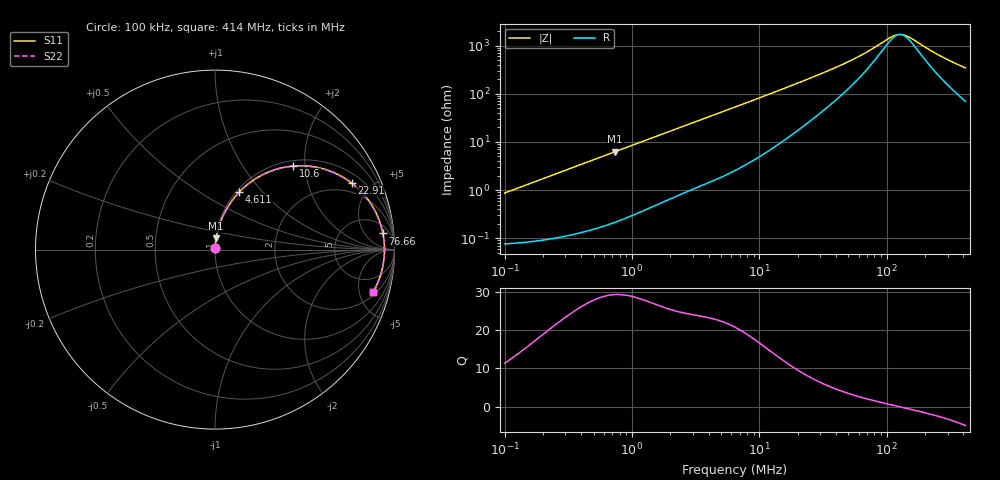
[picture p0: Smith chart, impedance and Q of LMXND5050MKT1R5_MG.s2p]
! LMXND5050MKT1R5_MG  S-PARAMETER MODEL  ( General Type )
! Model Generated by TAIYO YUDEN Corporation (http://www.ty-top.com)
! Version 1.0
! TAIYO YUDEN Control No. 191023NI43SB-FBB
! Copyright(c) 2019 TAIYO YUDEN CO.,LTD. All Rights Reserved.
! Product Description (link to TY-COMPAS)
! https://ds.yuden.co.jp/TYCOMPAS/or/detail?pn=LMXND5050MKT1R5NMG&u=M
! Products Name : Inductors
! Characteristics :
!  Inductance : 1.5 uH , SRF(min) : 86 MHz , DC Resistance(max) : 0.084 Ohm
!  Rated Current : Saturation :3800 mA , Temp Rise : 2200 mA
!  Case Size : 4.9 x 4.9 / 0.193 x 0.193 [mm/inch] , Thickness : 1.2 / 0.047 [mm/inch]
!  (Conditions: Temperature = 25 degC , DC Bias Current/Voltage = 0A / 0V)
! External Node Assignments :
!  1  o---GGG---o  2
! GND o---------o GND
! Frequency Range : 0.1MHz  -  413.982163MHz  [ 402 STEP ]
# MHz S RI R 50
! Freq[MHz].  S11 Real  S11 Imag  S21 Real  S21 Imag  S12 Real  S12 Imag  S22 Real  S22 Imag
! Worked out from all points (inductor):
!   401 points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, 100 kHz to 414 MHz, reference 50 ohm
!   read as one part in series: L = 1.38 uH near 104.3 kHz
!   highest Q = 29.2 at 738 kHz (marker M1), where L = 1.35 uH
!   self-resonance near 127.1 MHz
!   S11 on the Smith chart (normalised r, x): 100 kHz: 1.00, +0.02; 4.611 MHz: 1.03, +0.76; 10.6 MHz: 1.11, +1.74; 22.91 MHz: 1.45, +3.80; 76.66 MHz: 10, +15; 414 MHz: 2.39, -6.73
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0.1  0.000837 0.00864  0.9992 -0.00864  0.9992 -0.00864  0.000837 0.00864
0.403501  0.00251 0.0344  0.9975 -0.0344  0.9975 -0.0344  0.00251 0.0344
0.738033  0.00605 0.0623  0.994 -0.0623  0.994 -0.0623  0.00605 0.0623
1.628129  0.0232 0.1329  0.9768 -0.1329  0.9768 -0.1329  0.0232 0.1329
2.916605  0.0636 0.2241  0.9364 -0.2241  0.9364 -0.2241  0.0636 0.2241
4.611174  0.1364 0.3219  0.8636 -0.3219  0.8636 -0.3219  0.1364 0.3219
6.434145  0.2285 0.3965  0.7715 -0.3965  0.7715 -0.3965  0.2285 0.3965
10.60498  0.4348 0.4655  0.5652 -0.4655  0.5652 -0.4655  0.4348 0.4655
15.10885  0.6 0.4508  0.4 -0.4508  0.4 -0.4508  0.6 0.4508
22.91292  0.7606 0.3714  0.2394 -0.3714  0.2394 -0.3714  0.7606 0.3714
25.96183  0.7971 0.3404  0.2029 -0.3404  0.2029 -0.3404  0.7971 0.3404
34.74798  0.8614 0.2657  0.1386 -0.2657  0.1386 -0.2657  0.8614 0.2657
47.48609  0.904 0.1898  0.096 -0.1898  0.096 -0.1898  0.904 0.1898
60.96434  0.9243 0.1353  0.0757 -0.1353  0.0757 -0.1353  0.9243 0.1353
76.65542  0.9356 0.09  0.0644 -0.09  0.0644 -0.09  0.9356 0.09
104.7562  0.9431 0.0335  0.0569 -0.0335  0.0569 -0.0335  0.9431 0.0335
121.1928  0.9443 0.00821  0.0557 -0.00821  0.0557 -0.00821  0.9443 0.00821
129.0043  0.9444 -0.00256  0.0556 0.00256  0.0556 0.00256  0.9444 -0.00256
140.2084  0.9441 -0.0169  0.0559 0.0169  0.0559 0.0169  0.9441 -0.0169
155.5917  0.9431 -0.035  0.0569 0.035  0.0569 0.035  0.9431 -0.035
261.847  0.9253 -0.133  0.0747 0.133  0.0747 0.133  0.9253 -0.133
413.9822  0.8806 -0.237  0.1194 0.237  0.1194 0.237  0.8806 -0.237
